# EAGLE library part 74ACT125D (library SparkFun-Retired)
Quad Buffer with 3-State Outputs- ON Semi Conductor: Digikey P/N 74ACT125SC-ND
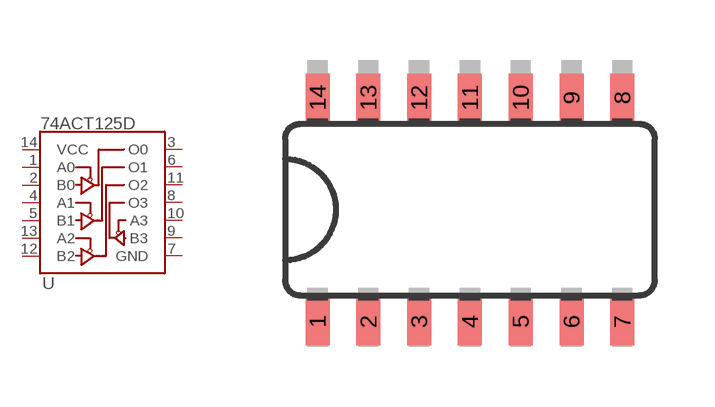
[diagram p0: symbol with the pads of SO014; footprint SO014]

Designator prefix -

## 74ACT125D  [SO014]
1  A0
2  B0
3  O0
4  A1
5  B1
6  O1
7  GND
8  O3
9  B3
10  A3
11  O2
12  B2
13  A2
14  VCC

## Footprint SO014 (pad centres in mm)
smd 0.6 x 1.2: 1 -3.175,-2.8; 2 -1.905,-2.8; 3 -0.635,-2.8; 4 0.635,-2.8; 5 1.905,-2.8; 6 3.175,-2.8; 7 4.445,-2.8; 8 4.445,2.8; 9 3.175,2.8; 10 1.905,2.8; 11 0.635,2.8; 12 -0.635,2.8; 13 -1.905,2.8; 14 -3.175,2.8

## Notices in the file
Licensing: Creative Commons ShareAlike 4.0 International - https://creativecommons.org/licenses/by-sa/4.0
Released under the Creative Commons Attribution Share-Alike 3.0 License
https://creativecommons.org/licenses/by-sa/3.0
http://creativecommons.org/licenses/by-sa/3.0
Creative Commons License summary- RETIRED.
